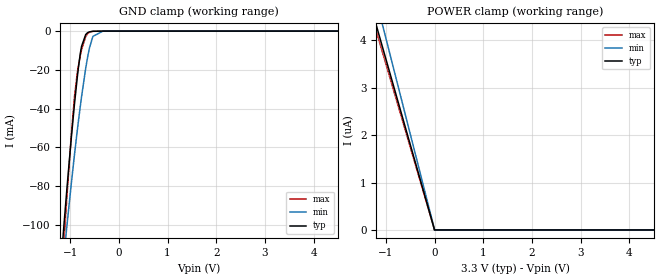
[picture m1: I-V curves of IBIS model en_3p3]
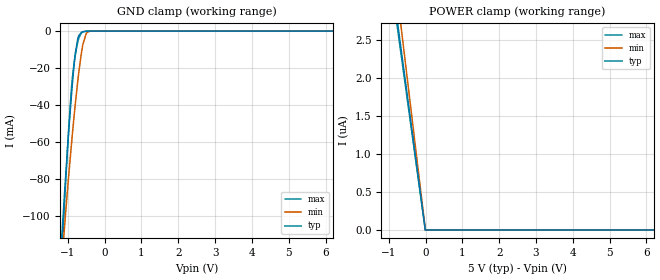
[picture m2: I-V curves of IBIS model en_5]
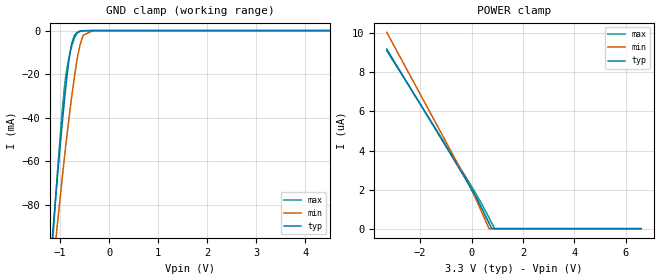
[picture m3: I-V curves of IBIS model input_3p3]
|Texas Instruments Incorporated
| ISO7821LLS High-Performance, 8000 VPK Reinforced Isolated Dual LVDS Buffer
| Marketing part#   Digital Voltage Range   Package-type   #pins
| ISO7821LLS   2.25V-5.5V   SOIC   16
[IBIS Ver]   4.1
[File name]   iso7821lls.ibs
[File Rev]   1.0
[Date]   10/21/2015
[Source]
| Texas Instruments Incorporated.
| Analog-eLab Design Center, HPA
| 12500 TI Blvd
| Dallas, TX -75243
[Notes]   Revision History:
| Rev 1.0: 10/21/2015
| - Initial version of the model
| - Model generated from simulations in SPECTRE
| - Model matched to SPICE simulation
| - C_comp although listed in numerical order of value are
|   obtained from varying PVT conditions. For PVT conditions for
|   each specific value refer the buffer description under
|   respective [Model]. IBIS model user is responsible for using
|   appropriate C_comp to simulate for Signal Integrity.
|* EXCEPTION:   *
|* - For models input_*,there will be leakage in power clamp/ground   *
|*   clamp IV tables because of resistors connected to pad.   *
|* - For models lvds_*,there will be leakage in IV tables because of   *
|*   driver switch arrangement   *
[Disclaimer]
| This model is designed as an aid for customers of Texas Instruments.
| TI and its licensors and suppliers make no warranties, either expressed
| or implied, with respect to this  model, including the warranties of
| merchantability or fitness for a particular purpose. The model is
| provided solely on an "as is" basis. The entire risk as to its quality
| and performance is with the customer.
[Copyright]
(C) Copyright 2015 Texas Instruments Incorporated.All rights reserved.
|   ISO7821LLSDW
[Component]   ISO7821LLSDW
[Manufacturer]   TI
[Package]   |16 SOIC  -  DW package
|   typ   min   max
R_pkg   0.23488   0.18142   0.33899
L_pkg   2.98751nH   2.67539nH   3.60953nH
C_pkg   0.09433pF   0.00463pF   0.13640pF
[Pin]  signal_name   model_name   R_pin   L_pin   C_pin
1   VCC1   power   0.26566   3.82128nH  0.41715pF
2   GND1   gnd   0.12519   3.78813nH  0.16384pF
3   INAP   input   0.18142   2.67539nH  0.12179pF
4   INAM   input   0.25612   3.03319nH  0.10465pF
5   OUTBM   lvds   0.22556   2.69927nH  0.12001pF
6   OUTBP   lvds   0.20725   2.71043nH  0.10107pF
7   EN1   en   0.21324   3.11387nH  0.00864pF
8   GND1   gnd   0.25706   3.76416nH  0.18155pF
9   GND2   gnd   0.08931   2.84540nH  0.10084pF
10   EN2   en   0.22039   3.56255nH  0.11986pF
11   INBP   input   0.33899   3.60953nH  0.10458pF
12   INBM   input   0.26965   3.01866nH  0.12171pF
13   OUTAM   lvds   0.22422   2.73387nH  0.13640pF
14   OUTAP   lvds   0.21197   2.71835nH  0.00463pF
15   GND2   gnd   0.22032   3.07227nH  0.02694pF
16   VCC2   power   0.14532   4.06977nH  0.02551pF
[Diff_pin]   inv_pin   vdiff   tdelay_typ   tdelay_min   tdelay_max
3   4   600mV   NA   NA   NA
6   5   NA   NA   NA   NA
11   12   600mV   NA   NA   NA
14   13   NA   NA   NA   NA
|   Model Selectors
[Model Selector] input
input_3p3 3.3V  digital input
input_5   5V   digital input
[Model Selector] en
en_3p3   3.3V   digital input
en_5   5V   digital input
[Model Selector] lvds
lvds_3p3 3.3V   digital output
lvds_5   5V   digital output
| Models and submodels in the file (6): en_3p3 (Input), en_5 (Input), input_3p3 (Input), input_5 (Input), lvds_3p3 (3-state), lvds_5 (3-state)
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|   en_3p3 Model
[Model]   en_3p3
Model_type   Input
Vinl = 0.8
Vinh = 2
|   typ   min   max
|   (nom PVT)   (fast PVT)   (slow PVT)
C_comp   5.145e-12   5.099e-12   5.287e-12
| Where nom  PVT is Nominal Process, 3.3V, 27C
|   Fast PVT is Strong Process,  3.6V, -55C
|   Slow PVT is Weak Process,   3V, 150C
[Voltage Range]   3.3   3   3.6
|Junction Temperature
[Temperature Range]   27   150   -55
[Power Clamp Reference]   3.3   3   3.6
[GND Clamp Reference]   0   0   0
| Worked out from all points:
|   GND clamp passes 1 mA (typ) near -0.65 V on its own axis
[GND Clamp]
|   Voltage   I(typ)   I(min)   I(max)
-3.3V     -929.9mA   -786.9mA   -1.112A
-1.208V   -125.8mA   -136.9mA   -141.1mA
-1.126V   -99.36mA   -115.3mA   -108mA
-1.068V   -81.64mA   -100.8mA   -85.93mA
-915mV    -38.49mA   -64.49mA   -34.73mA
-855.6mV  -24.14mA   -51.61mA   -21.9mA
-765.6mV  -7.846mA   -33.74mA   -9.556mA
-681mV    -1.778mA   -19.2mA    -2.852mA
-603mV    -400.9uA   -8.586mA   -571.6uA
-534mV    -100.9uA   -2.759mA   -113.2uA
-330mV    -13.5uA    -29.87uA   -13.86uA
6.6V      0A         0A         0A
[POWER Clamp]
|   Voltage   I(typ)   I(min)   I(max)
-3.3V     11.89uA    13.33uA    11.55uA
-1.234V   4.439uA    4.978uA    4.31uA
-1.023V   3.679uA    4.126uA    3.572uA
-6mV      0A         16.89nA    0A
-3.3mV    0A         0A         0A
6.6V      0A         0A         0A
|   en_5 Model
[Model]   en_5
Model_type   Input
Vinl = 0.8
Vinh = 2
|   typ   min   max
|   (nom PVT)   (fast PVT)   (slow PVT)
C_comp   5.145e-12   5.099e-12   5.287e-12
| Where nom  PVT is Nominal Process, 5V, 27C
|   Fast PVT is Strong Process,  5.5V, -55C
|   Slow PVT is Weak Process,   4.5V, 150C
[Voltage Range]   5   4.5   5.5
|Junction Temperature
[Temperature Range]   27   150   -55
[Power Clamp Reference]   5   4.5   5.5
[GND Clamp Reference]   0   0   0
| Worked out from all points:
|   GND clamp passes 1 mA (typ) near -0.64 V on its own axis
[GND Clamp]
|   Voltage   I(typ)   I(min)   I(max)
-5V       -1.629A    -1.369A    -1.924A
-1.161V   -110.2mA   -124.2mA   -121.4mA
-1.067V   -80.98mA   -100.3mA   -85.03mA
-968.5mV  -52.31mA   -76.37mA   -50.1mA
-897mV    -33.53mA   -60.18mA   -29.78mA
-870mV    -27.04mA   -54.34mA   -24.15mA
-795mV    -11.87mA   -39.05mA   -12.77mA
-730mV    -4.164mA   -27.06mA   -5.982mA
-594.5mV  -332.9uA   -7.503mA   -455.7uA
-500mV    -57.82uA   -1.284mA   -57.52uA
-351.5mV  -20.04uA   -47.36uA   -20.7uA
10V       0A         0A         0A
[POWER Clamp]
|   Voltage   I(typ)   I(min)   I(max)
-5V       18.02uA    20.21uA    17.5uA
-1.067V   3.832uA    4.3uA      3.72uA
-500mV    1.786uA    2.009uA    1.733uA
-6mV      0A         12.17nA    0A
-5mV      0A         0A         0A
10V       0A         0A         0A
|   input_3p3 Model
[Model]   input_3p3
Model_type   Input
Vinl = 0.8
Vinh = 2
|   typ   min   max
|   (nom PVT)   (fast PVT)   (slow PVT)
C_comp   3.961e-12   3.930e-12   4.057e-12
| Where nom  PVT is Nominal Process, 3.3V, 27C
|   Fast PVT is Strong Process,  3.6V, -55C
|   Slow PVT is Weak Process,   3V, 150C
[Voltage Range]   3.3   3   3.6
|Junction Temperature
[Temperature Range]   27   150   -55
[Power Clamp Reference]   3.3   3   3.6
[GND Clamp Reference]   0   0   0
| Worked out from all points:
|   GND clamp passes 1 mA (typ) near -0.66 V on its own axis
[GND Clamp]
|   Voltage   I(typ)   I(min)   I(max)
-3.3V     -797mA     -692.8mA   -932.5mA
-1.162V   -96.29mA   -113.4mA   -100.6mA
-1.089V   -76.44mA   -96.71mA   -76.55mA
-1.054V   -67.05mA   -88.76mA   -65.26mA
-970.8mV  -46.04mA   -70.72mA   -40.65mA
-891mV    -27.57mA   -54.23mA   -22.11mA
-821.7mV  -14.01mA   -40.83mA   -12.7mA
-762.3mV  -5.878mA   -30.18mA   -7.052mA
-636mV    -590.3uA   -11.15mA   -910.3uA
-531mV    -70.89uA   -2.138mA   -78.36uA
-330mV    -7.807uA   -20.99uA   -7.825uA
6.6V      0A         0A         0A
[POWER Clamp]
|   Voltage   I(typ)   I(min)   I(max)
-3.3V     9.193uA    10.05uA    9.116uA
-111mV    2.273uA    2.267uA    2.407uA
189mV     1.58uA     1.463uA    1.745uA
681mV     290nA      0A         558.6nA
788.7mV   0A         0A         282.6nA
897.6mV   0A         0A         0A
6.6V      0A         0A         0A
